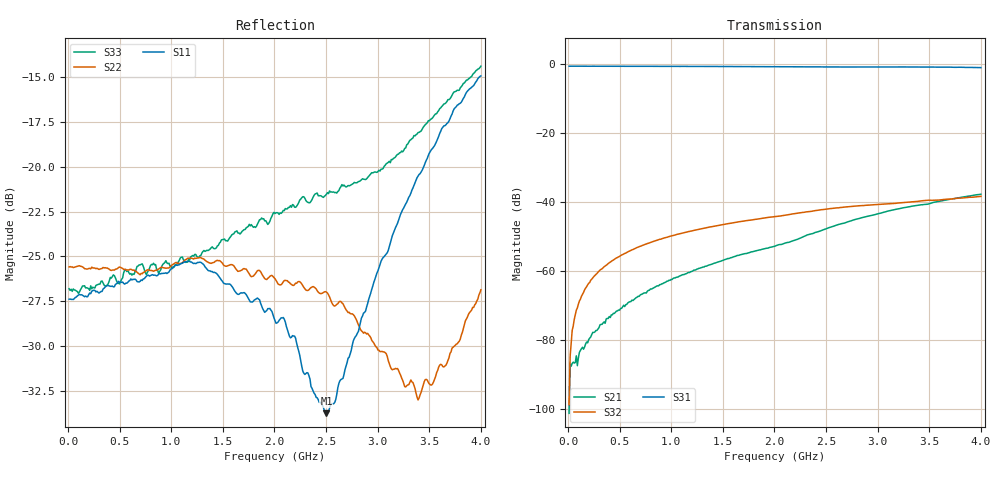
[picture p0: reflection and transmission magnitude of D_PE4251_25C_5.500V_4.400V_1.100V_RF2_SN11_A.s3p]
! Device ID: PE4251_SoldCshunt_081809
! Dir: c:\Test Bench Repositories\Bench_Software_CVI_Version_8\trunk\PSC 4Port_VNA Bench\datalog\4250\TEST\PE4251_SoldCshunt_081809\25C\5p500000\RF2
! Serial: 11
! Insertion: A
! Temp: 25C
! VDD: 5.500
! Control_Hi: 80.000
! Control_Lo: 20.000
! Logic State: RF2
! Port 1: RFC
! Port 2: RF1
! Port 3: RF2
! V1 = 1.10
! V2 = 1.10
! V3 = 1.10
! IDD: 6.953680e-05
! FILE NAME
! DATE 08/18/09  20:15
! CORRECTED  DATA
#  Hz  S  RI  R  50.00
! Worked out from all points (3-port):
!   401 points, 10 MHz to 4 GHz, reference 50 ohm
!   strongest paths, dB at 10 MHz, 1.008 GHz, 2.005 GHz, 3.002 GHz, 4 GHz:
!     S31: -0.6, -0.6, -0.7, -0.8, -1.0
!     S32: -98.8, -49.8, -44.2, -40.7, -38.3
!     S21: -101.3, -62.5, -52.8, -43.4, -37.7
!   lowest |S11| = -33.7 dB at 2.504 GHz (marker M1), VSWR 1.04, Z = 50.5 - j2 ohm
!   |S11| at or under -10 dB: start of sweep to end of sweep
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1e7  0.0428 -0.000554  4.58e-06 -5.47e-05  0.9372 -0.00287
     5.84e-06 -6.29e-06  0.0526 -0.000806  5.79e-05 -7.06e-05
     0.9381 -0.00486  -2.76e-06 1.11e-05  0.0457 0.000491
9.9775e7  0.0438 0.00176  1.49e-05 -5.3e-05  0.9381 -0.0353
          1.86e-05 -5.14e-05  0.0529 -0.000853  5.09e-05 0.00032
          0.939 -0.0352  4.07e-05 0.000327  0.0444 9.21e-05
1.79575e8  0.0434 0.00236  2.19e-07 -9.53e-05  0.9361 -0.0628
           1.07e-06 -9.28e-05  0.0518 -0.00101  5.78e-05 0.000589
           0.9364 -0.0629  5.01e-05 0.00059  0.046 0.000831
2.99275e8  0.0444 0.00278  -4.46e-05 -0.000141  0.932 -0.1042
           -5.18e-05 -0.000141  0.0517 -0.0025  7.77e-05 0.00098
           0.9321 -0.1034  9.02e-05 0.000989  0.0471 -0.00104
4.78825e8  0.0474 0.00114  -0.000154 -0.000215  0.9213 -0.1644
           -0.000152 -0.000215  0.0518 -0.00499  0.000144 0.00157
           0.9214 -0.1636  0.000134 0.00156  0.0472 -0.00464
1.037425e9  0.0517 -0.0116  -0.000723 -0.000325  0.8686 -0.3428
            -0.000725 -0.000319  0.0525 -0.0122  0.000477 0.0033
            0.8692 -0.3423  0.000488 0.0033  0.0523 -0.0107
2.005e9  0.0349 -0.0131  -0.00224 -0.000432  0.7 -0.5994
         -0.00225 -0.000433  0.0483 -0.00681  0.00112 0.00606
         0.701 -0.5989  0.00112 0.00606  0.0672 -0.0311
2.50375e9  0.00559 -0.0198  -0.00403 -0.000859  0.5904 -0.6967
           -0.00402 -0.000863  0.0447 0.000458  0.00151 0.00775
           0.5931 -0.6965  0.00152 0.00777  0.0536 -0.0644
3.391525e9  -0.0858 -0.0388  -0.00899 0.000912  0.3567 -0.8394
            -0.00897 0.00092  0.0128 0.0184  0.00215 0.01
            0.3581 -0.8402  0.00214 0.0101  -0.0248 -0.1219
4e9  -0.1768 -0.0273  -0.0126 0.0035  0.1435 -0.8846
     -0.0125 0.00348  -0.0271 0.0364  0.00225 0.0118
     0.1448 -0.884  0.00225 0.0119  -0.1312 -0.138
